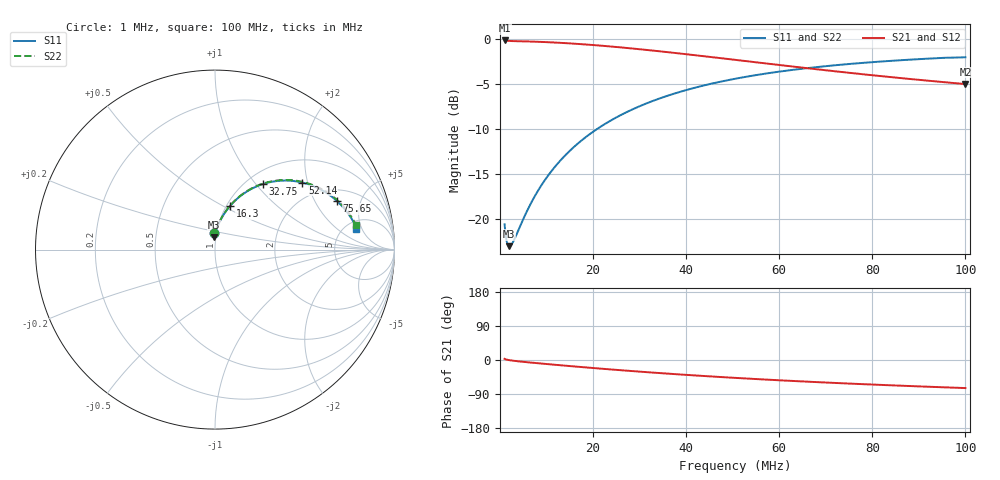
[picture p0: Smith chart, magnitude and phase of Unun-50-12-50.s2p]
! ListType=Log
!!Unun 2 Unun 50-12.5-50
# MHZ S RI R 50
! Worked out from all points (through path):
!   100 points, 1 MHz to 100 MHz, reference 50 ohm
!   highest |S21| = -0.12 dB at 1 MHz (marker M1); lowest = -5.0 dB at 100 MHz (marker M2)
!   group delay of S21, straight-line fit = 2.32 ns
!   lowest |S11| = -23.1 dB at 2.009 MHz (marker M3), VSWR 1.15, Z = 48.7 + j6.84 ohm
!   |S11| at or under -10 dB: start of sweep to 20.86 MHz
!   |S22| runs from -23.1 to -2.0 dB; largest |S21 - S12| = 0.0023
!   S11 on the Smith chart (normalised r, x): 1 MHz: 0.97, +0.18; 16.3 MHz: 1.04, +0.54; 32.75 MHz: 1.19, +1.09; 52.14 MHz: 1.55, +1.86; 75.65 MHz: 2.64, +3.07; 100 MHz: 6.19, +3.92
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1  -0.00821 0.0928  0.9846 0.0532  0.9846 0.0531  -0.00825 0.0928
1.204503  -0.00751 0.0817  0.9845 0.0346  0.9845 0.0346  -0.00754 0.0817
1.450829  -0.00769 0.0745  0.9832 0.0183  0.9832 0.0183  -0.00774 0.0744
1.747528  -0.00795 0.0707  0.9816 0.00375  0.9816 0.00373  -0.00798 0.0706
2.009233  -0.00792 0.0698  0.9804 -0.00652  0.9804 -0.00652  -0.00796 0.0698
2.782559  -0.00657 0.0736  0.9776 -0.0302  0.9777 -0.0302  -0.00657 0.0736
6.428073  0.00937 0.1184  0.9663 -0.1101  0.9663 -0.1101  0.00924 0.1184
8.902151  0.0241 0.1517  0.9547 -0.1572  0.9547 -0.1572  0.0238 0.1517
12.32847  0.0488 0.196  0.9333 -0.2177  0.9333 -0.2177  0.0484 0.1961
16.29751  0.0834 0.2426  0.9019 -0.2815  0.9018 -0.2815  0.0827 0.2429
17.8865  0.0988 0.2596  0.8875 -0.3053  0.8875 -0.3053  0.0979 0.26
21.54435  0.1368 0.2948  0.8516 -0.3556  0.8516 -0.3556  0.1356 0.2953
24.77076  0.1729 0.3207  0.8172 -0.3951  0.8172 -0.3951  0.1714 0.3215
32.74549  0.2673 0.3652  0.7257 -0.4733  0.7257 -0.4733  0.265 0.3669
34.30469  0.286 0.3708  0.7073 -0.4856  0.7073 -0.4856  0.2836 0.3726
43.28761  0.3918 0.3847  0.6025 -0.5387  0.6025 -0.5387  0.3887 0.3879
52.14008  0.4871 0.3734  0.5059 -0.5675  0.5059 -0.5675  0.4834 0.3782
59.94843  0.5611 0.3484  0.4287 -0.5784  0.4287 -0.5784  0.5571 0.3548
68.92612  0.6334 0.3075  0.3506 -0.5796  0.3506 -0.5796  0.6294 0.3158
75.64633  0.679 0.2712  0.2992 -0.5752  0.2992 -0.5752  0.6751 0.2809
86.9749  0.7402 0.2031  0.2247 -0.5618  0.2247 -0.5618  0.7368 0.2152
100  0.7856 0.1168  0.1545 -0.5415  0.1567 -0.5421  0.7852 0.1353
